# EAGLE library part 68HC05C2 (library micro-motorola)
MICROCONTROLLER/MEMORY DEVICE
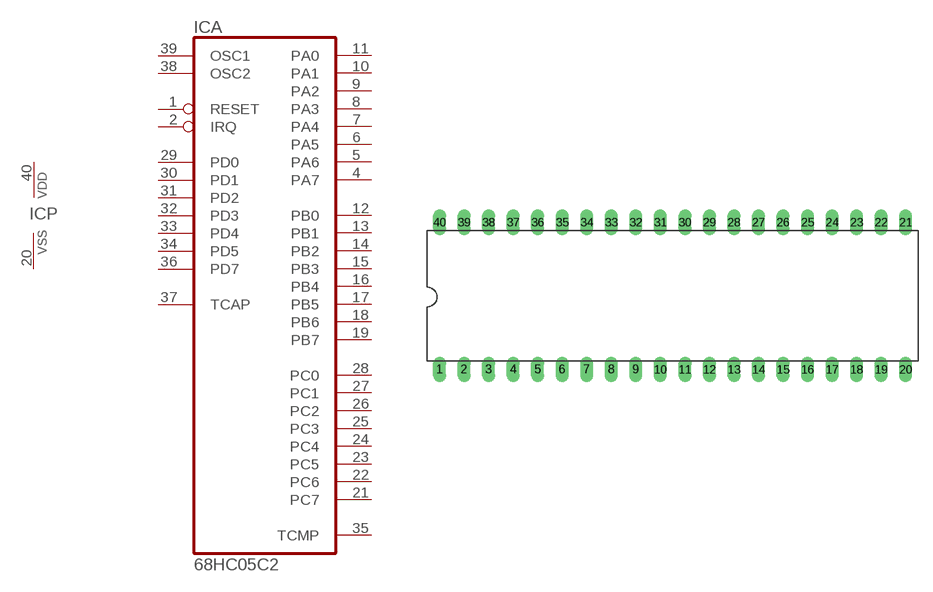
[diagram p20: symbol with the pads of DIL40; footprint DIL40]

Designator prefix IC; gates A=68HC05C2 P=VSSVDD

## 68HC05C2 (MF: MOTOROLA; MPN: MC68HC705SR3CPE; OC_FARNELL: 1749029; OC_NEWARK: 40K7346)  [DIL40]
1  A:RESET  in
2  A:IRQ  in
4  A:PA7
5  A:PA6
6  A:PA5
7  A:PA4
8  A:PA3
9  A:PA2
10  A:PA1
11  A:PA0
12  A:PB0
13  A:PB1
14  A:PB2
15  A:PB3
16  A:PB4
17  A:PB5
18  A:PB6
19  A:PB7
20  P:VSS  pwr
21  A:PC7
22  A:PC6
23  A:PC5
24  A:PC4
25  A:PC3
26  A:PC2
27  A:PC1
28  A:PC0
29  A:PD0  in
30  A:PD1  in
31  A:PD2  in
32  A:PD3  in
33  A:PD4  in
34  A:PD5  in
35  A:TCMP  out
36  A:PD7  in
37  A:TCAP  in
38  A:OSC2  pas
39  A:OSC1  in
40  P:VDD  pwr

## Footprint DIL40 (pad centres in mm)
Dual In Line Package
drill 0.813 long: 1 -24.13,-7.62; 2 -21.59,-7.62; 3 -19.05,-7.62; 4 -16.51,-7.62; 5 -13.97,-7.62; 6 -11.43,-7.62; 7 -8.89,-7.62; 8 -6.35,-7.62; 9 -3.81,-7.62; 10 -1.27,-7.62; 11 1.27,-7.62; 12 3.81,-7.62; 13 6.35,-7.62; 14 8.89,-7.62; 15 11.43,-7.62; 16 13.97,-7.62; 17 16.51,-7.62; 18 19.05,-7.62; 19 21.59,-7.62; 20 24.13,-7.62; 21 24.13,7.62; 22 21.59,7.62; 23 19.05,7.62; 24 16.51,7.62; 25 13.97,7.62; 26 11.43,7.62; 27 8.89,7.62; 28 6.35,7.62; 29 3.81,7.62; 30 1.27,7.62; 31 -1.27,7.62; 32 -3.81,7.62; 33 -6.35,7.62; 34 -8.89,7.62; 35 -11.43,7.62; 36 -13.97,7.62; 37 -16.51,7.62; 38 -19.05,7.62; 39 -21.59,7.62; 40 -24.13,7.62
